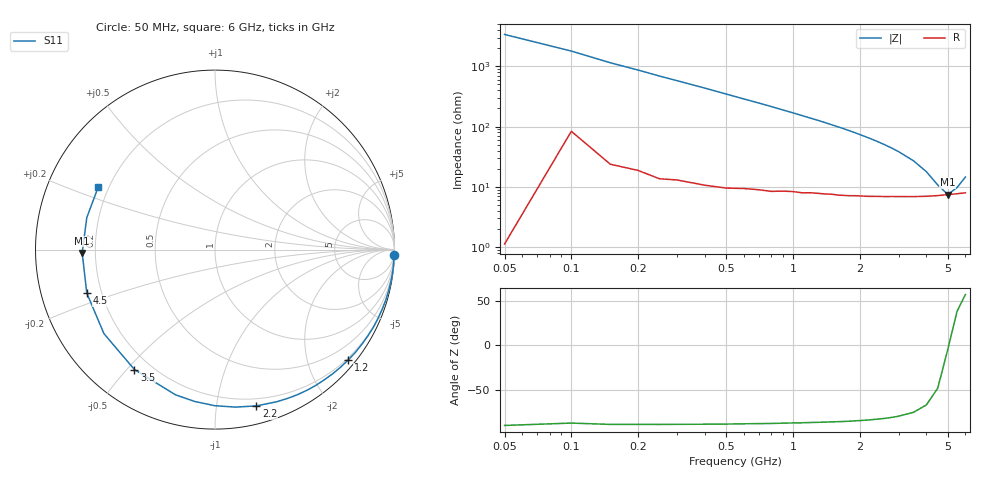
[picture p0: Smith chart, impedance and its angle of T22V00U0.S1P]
! SIEMENS Discrete & RF Semiconductors
! BAS70-04W
! Si Schottky Diode in SOT323
! VR = 2 V
! S-Parameters:  November  1997
# GHz  S  MA  R  50
!  f  S11
! GHz  MAG  ANG
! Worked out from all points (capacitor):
!   34 points, 50 MHz to 6 GHz, reference 50 ohm
!   read as one part to ground: C = 926 fF near 50 MHz
!   lowest |Z| = 7.49 ohm at 5 GHz (marker M1)
!   series resonance near 5.045 GHz, so ESL is about 1.1 nH
!   S11 on the Smith chart (normalised r, x): 50 MHz: 0, -67; 1.2 GHz: 0.16, -2.76; 2.2 GHz: 0.14, -1.29; 3.5 GHz: 0.14, -0.52; 4.5 GHz: 0.14, -0.16; 6 GHz: 0.16, +0.24
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0.05  1 -1.7
0.1  0.9974 -3.2
0.15  0.9982 -5.0
0.25  0.9971 -8.3
0.4  0.9944 -13.1
0.5  0.9922 -16.4
0.6  0.989 -19.7
0.8  0.9828 -26.2
1  0.9734 -32.9
1.1  0.9694 -36.3
1.2  0.9636 -39.7
1.3  0.9587 -43.0
1.4  0.9534 -46.5
1.6  0.9422 -53.5
1.8  0.9294 -60.6
1.9  0.922 -64.2
2  0.9149 -67.9
2.2  0.9007 -75.2
2.4  0.8849 -82.6
2.6  0.8697 -90.1
2.8  0.8536 -97.6
3  0.8385 -105.2
3.5  0.805 -123.9
4  0.7759 -142.9
4.5  0.7543 -161.3
5  0.7401 -178.6
5.5  0.7362 166.0
6  0.738 151.9
